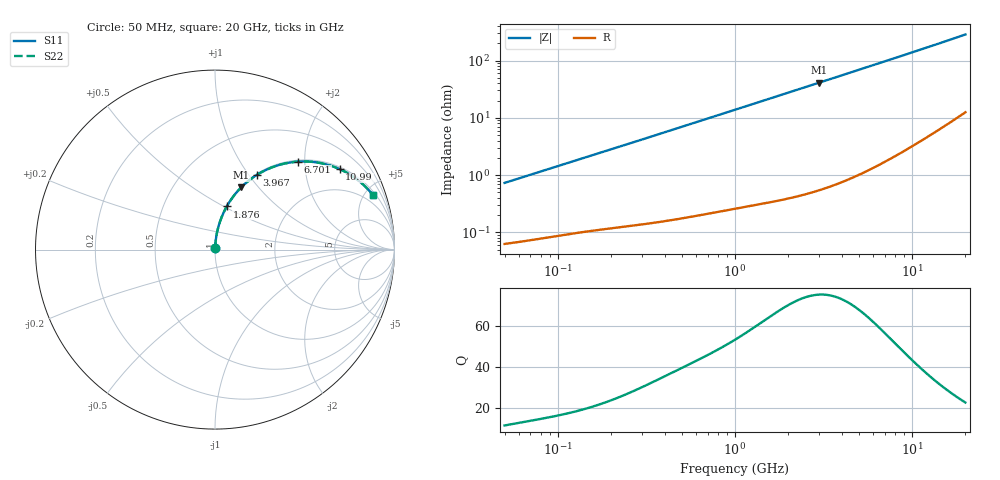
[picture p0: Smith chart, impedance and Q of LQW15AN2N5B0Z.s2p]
!Murata Part Number: LQW15AN2N5B0Z
!These Parameters are Measured in Series Mode Connection
!  o--[Z]--o
!Port1  Port2
!  o-------o
!Freq. Start=50[MHz] Stop=20[GHz], 401[Steps]
# Hz S RI R 50
!Freq.(Hz) S11(Real) S11(Imag) S21(Real) S21(Imag) S12(Real) S12(Imag) S22(Real) S22(Imag)
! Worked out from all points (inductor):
!   401 points, 50 MHz to 20 GHz, reference 50 ohm
!   read as one part in series: L = 2.31 nH near 51.52 MHz
!   highest Q = 75.6 at 2.985 GHz (marker M1), where L = 2.19 nH
!   S11 on the Smith chart (normalised r, x): 50 MHz: 1.00, +0.01; 1.876 GHz: 1.01, +0.52; 3.967 GHz: 1.01, +1.09; 6.701 GHz: 1.03, +1.85; 10.99 GHz: 1.08, +3.05; 20 GHz: 1.25, +5.70
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5e7  0.000682 0.00728  0.9993 -0.00728  0.9993 -0.00728  0.000682 0.00728
1.364002e8  0.00138 0.0193  0.9986 -0.0193  0.9986 -0.0193  0.00138 0.0193
2.33884e8  0.00233 0.0327  0.9977 -0.0327  0.9977 -0.0327  0.00233 0.0327
3.721004e8  0.00419 0.0517  0.9958 -0.0517  0.9958 -0.0517  0.00419 0.0517
6.285508e8  0.0095 0.0863  0.9905 -0.0863  0.9905 -0.0863  0.0095 0.0863
1e9  0.0212 0.135  0.9788 -0.135  0.9788 -0.135  0.0212 0.135
1.369645e9  0.0372 0.1813  0.9628 -0.1813  0.9628 -0.1813  0.0372 0.1813
1.875929e9  0.0656 0.2404  0.9344 -0.2404  0.9344 -0.2404  0.0656 0.2404
2.279204e9  0.0927 0.2833  0.9073 -0.2833  0.9073 -0.2833  0.0927 0.2833
2.728004e9  0.1267 0.3261  0.8733 -0.3261  0.8733 -0.3261  0.1267 0.3261
2.98453e9  0.1475 0.348  0.8525 -0.348  0.8525 -0.348  0.1475 0.348
3.466789e9  0.1885 0.3845  0.8115 -0.3845  0.8115 -0.3845  0.1885 0.3845
3.967106e9  0.2325 0.4157  0.7675 -0.4157  0.7675 -0.4157  0.2325 0.4157
5.273168e9  0.3473 0.4687  0.6527 -0.4687  0.6527 -0.4687  0.3473 0.4687
6.701223e9  0.4612 0.49  0.5388 -0.49  0.5388 -0.49  0.4612 0.49
7.442007e9  0.5131 0.4907  0.4869 -0.4907  0.4869 -0.4907  0.5131 0.4907
9.041845e9  0.6078 0.4778  0.3922 -0.4778  0.3922 -0.4778  0.6078 0.4778
1.098561e10  0.6949 0.4482  0.3051 -0.4482  0.3051 -0.4482  0.6949 0.4482
1.276073e10  0.7537 0.4169  0.2463 -0.4169  0.2463 -0.4169  0.7537 0.4169
1.482269e10  0.8041 0.3809  0.1959 -0.3809  0.1959 -0.3809  0.8041 0.3809
1.747767e10  0.8498 0.3387  0.1502 -0.3387  0.1502 -0.3387  0.8498 0.3387
2e10  0.88 0.3037  0.12 -0.3037  0.12 -0.3037  0.88 0.3037
